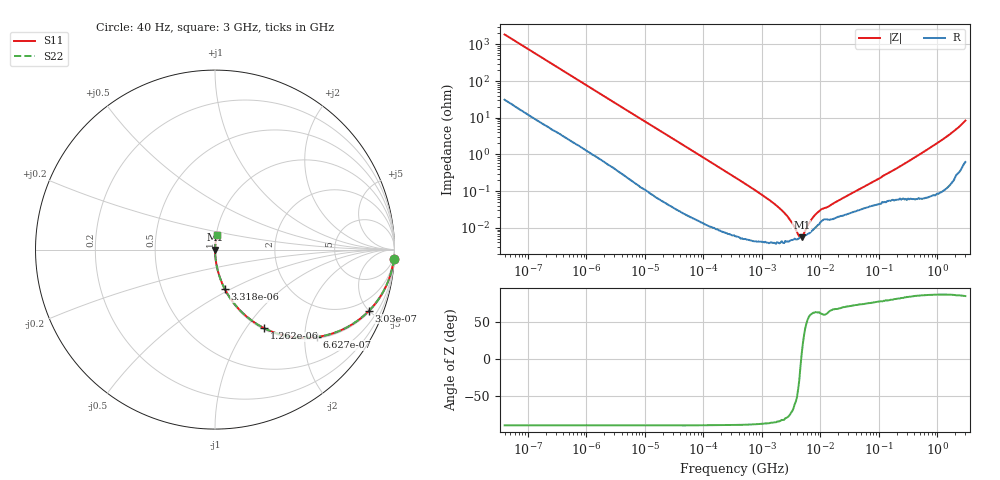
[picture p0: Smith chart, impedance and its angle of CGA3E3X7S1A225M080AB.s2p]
! S-parameter Generated by TDK Corporation
! Copyright(C) 2015 TDK Corporation.
! All Rights Reserved.
! TDK P/N: CGA3E3X7S1A225M080AB (Multilayer Ceramic Chip Capacitors)
! Property: C=2.2uF
! Size(LxWxT): 1.6x0.8x0.8mm, 0.063x0.031x0.031inches
! Model Type: s2p (Touchstone File Format Version 1.0)
! Frequency: DC=Yes Start=0.00004MHz Stop=3000MHz 396points Log-sweep
! Note: This model was converted from impedance.
! Model Generated on Jun. 23, 2015
! Hash(MD5):
! Port Assignments:
!  1 ---| |--- 2
! Applicable Conditions:
!  Temperature = 25 degC
!  DC Bias Voltage = 0 V
!  Small Signal Operation
! Terms and conditions regarding TDK Simulation Models
! (1)This simulation model is being provided solely for informational purposes. Please refer to the specifications of the products in terms of detailed characteristics of such products.
! (2)In no event shall TDK Corporation of any of its subsidiaries be liable for any loss or damage arising, directly or indirectly,
!  From any information contained in this simulation model, including, but not limited to loss or damages arising from any inaccuracies, omissions or errors in connection with such information.
! (3)Any and all copyrights on this simulation model are owned by TDK Corporation.
!  Duplication or redistribution of this simulation model without prior written permission from TDK Corporation is prohibited.
! (4)This simulation model is subject to any modification or change without any prior notice.
! (5)Neither TDK Corporation nor any of its subsidiaries shall make any warranty, express or implied,
!  Including but not limited to the correctness, implied warranties of merchantability and fitness for a particular purpose with respect to this simulation models.
! (6)The use of this simulation model shall be deemed to have consented to the terms and conditions hereof.
# MHz S MA R 50
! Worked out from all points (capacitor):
!   395 points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, 40 Hz to 3 GHz, reference 50 ohm
!   read as one part in series: C = 2.13 uF near 41.88 Hz
!   lowest |Z| = 5.52 mohm at 4.774 MHz (marker M1)
!   series resonance near 4.679 MHz, so ESL is about 540 pH
!   S11 on the Smith chart (normalised r, x): 40 Hz: 2, -37; 303 Hz: 1.08, -5.01; 662.7 Hz: 1.04, -2.31; 1.262 kHz: 1.02, -1.22; 3.318 kHz: 1.01, -0.47; 3 GHz: 1.01, +0.17
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4e-05  0.9977 -3.1  0.05344 86.0  0.05344 86.0  0.9977 -3.1
0.0001152847  0.9861 -8.7  0.1508 80.4  0.1508 80.4  0.9861 -8.7
0.0003030459  0.9236 -21.6  0.3684 67.4  0.3684 67.4  0.9236 -21.6
0.000662667  0.7497 -40.5  0.6495 48.6  0.6495 48.6  0.7497 -40.5
0.000834128  0.671 -46.9  0.7304 42.1  0.7304 42.1  0.671 -46.9
0.001262176  0.5169 -57.9  0.8476 31.1  0.8476 31.1  0.5169 -57.9
0.001999837  0.3592 -68.0  0.9274 21.0  0.9274 21.0  0.3592 -68.0
0.003317849  0.2284 -75.9  0.97 13.2  0.97 13.2  0.2284 -75.9
0.006928769  0.1135 -82.7  0.9919 6.5  0.9919 6.5  0.1135 -82.7
0.01739424  0.04624 -86.6  0.9983 2.7  0.9983 2.7  0.04624 -86.6
0.3464102  0.002386 -88.4  0.9999 0.1  0.9999 0.1  0.002386 -88.4
1.734411  0.0004165 -85.0  1 0.0  1 0.0  0.0004165 -85.0
2.748062  0.0002036 -78.0  1 0.0  1 0.0  0.0002036 -78.0
3.622024  0.0001043 -60.8  0.9999 0.0  0.9999 0.0  0.0001043 -60.8
4.773931  5.523e-05 7.3  0.9999 -0.0  0.9999 -0.0  5.523e-05 7.3
5.738865  9.626e-05 48.3  0.9999 -0.0  0.9999 -0.0  9.626e-05 48.3
7.22376  0.0001794 62.2  0.9999 -0.0  0.9999 -0.0  0.0001794 62.2
10.4391  0.0003227 61.8  0.9998 -0.0  0.9998 -0.0  0.0003227 61.8
13.75903  0.0003814 64.1  0.9998 -0.0  0.9998 -0.0  0.0003814 64.1
150.6385  0.003236 80.0  0.9994 -0.2  0.9994 -0.2  0.003236 80.0
1251.294  0.02621 86.3  0.9986 -1.5  0.9986 -1.5  0.02621 86.3
3000  0.08299 81.0  0.9904 -4.7  0.9904 -4.7  0.08299 81.0
